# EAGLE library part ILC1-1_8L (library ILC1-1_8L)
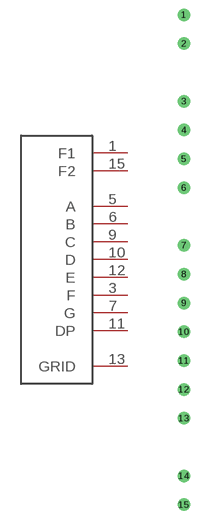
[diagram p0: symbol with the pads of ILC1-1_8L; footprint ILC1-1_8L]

Designator prefix -

## ILC1-1_8L  [ILC1-1_8L]
1  F1
3  F
5  A
6  B
7  G
9  C
10  D
11  DP
12  E
13  GRID
15  F2

## Footprint ILC1-1_8L (pad centres in mm)
drill 1.2 pad 2.2: 1 0,86.36; 2 0,81.28; 3 0,71.12; 4 0,66.04; 5 0,60.96; 6 0,55.88; 7 0,45.72; 8 0,40.64; 9 0,35.56; 10 0,30.48; 11 0,25.4; 12 0,20.32; 13 0,15.24; 14 0,5.08; 15 0,0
